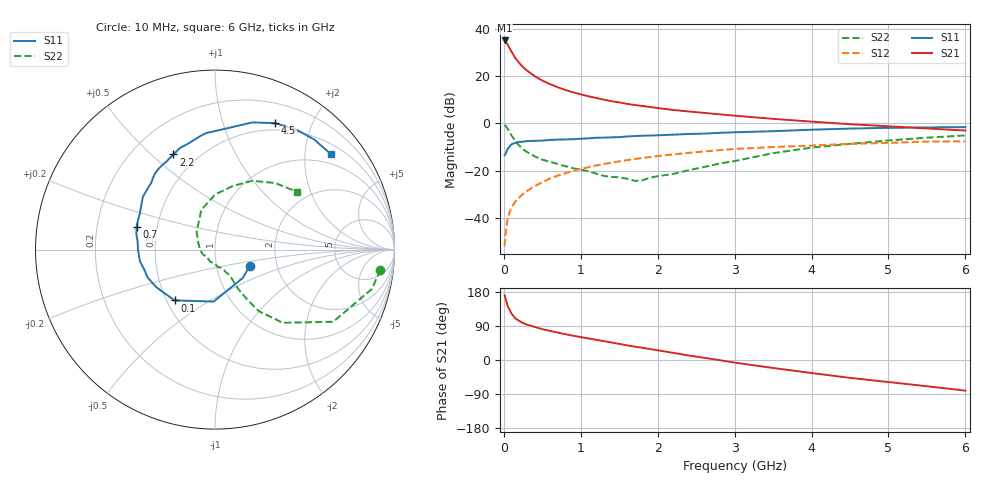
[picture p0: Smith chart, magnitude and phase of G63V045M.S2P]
! SIEMENS Small Signal Semiconductors
! BFG193
! Si NPN RF Bipolar Junction Transistor in SOT223
! VCE = 3 V  IC = 45 mA
! Common Emitter S-Parameters:  August  1996
# GHz  S  MA  R  50
!  f  S11  S21  S12  S22
! GHz  MAG  ANG  MAG  ANG  MAG  ANG  MAG  ANG
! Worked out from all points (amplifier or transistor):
!   36 points, 10 MHz to 6 GHz, reference 50 ohm
!   highest |S21| = 35.2 dB at 10 MHz (marker M1)
!   |S21| within 3 dB of that: start of sweep to 70.25 MHz
!   unconditionally stable (mu >= 1): 419.4 MHz to 2.427 GHz
!   at 250 MHz: K = 0.91, MSG = 26.9 dB, |S12| = -29.9 dB
!   at 1.4 GHz: K = 1.05, MAG = 11.7 dB, |S12| = -16.7 dB
!   at 6 GHz: K = 0.90, MSG = 2.3 dB, |S12| = -7.6 dB
!   S11 on the Smith chart (normalised r, x): 10 MHz: 1.45, -0.28; 100 MHz: 0.55, -0.36; 700 MHz: 0.38, +0.12; 2.2 GHz: 0.37, +0.59; 4.5 GHz: 0.42, +1.50; 6 GHz: 0.73, +2.60
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0.01  0.2138 -25.1  57.66 171.1  0.0025 82.6  0.9279 -7.0
0.02  0.2213 -45.4  55.79 163.3  0.0042 82.5  0.9011 -14.1
0.05  0.2896 -91.5  46.95 142.3  0.0099 70.2  0.7717 -31.4
0.1  0.3617 -128.5  33.24 122.4  0.0169 66.5  0.5558 -47.2
0.15  0.3886 -147.4  24.41 109.9  0.022 65.3  0.4198 -54.6
0.2  0.4062 -157.5  19.25 103.1  0.0269 66.3  0.3408 -56.9
0.25  0.4106 -165.1  15.7 97.6  0.0321 67.2  0.2828 -58.5
0.3  0.423 -170.8  13.27 93.4  0.037 68.6  0.25 -59.5
0.4  0.4284 -179.2  10.11 87.3  0.0468 68.5  0.2004 -59.9
0.5  0.4342 173.6  8.132 81.4  0.0568 67.6  0.171 -60.1
0.6  0.4475 168.5  6.834 76.8  0.0679 66.6  0.154 -61.6
0.7  0.4551 163.9  5.876 72.3  0.0781 65.5  0.1385 -64.4
0.9  0.4638 154.8  4.587 64.1  0.0991 61.8  0.1125 -68.9
1.1  0.4844 147.4  3.776 56.9  0.1184 58.3  0.0971 -80.4
1.3  0.5017 140.5  3.203 49.6  0.1384 54.2  0.0774 -92.2
1.6  0.5296 130.6  2.61 38.7  0.1669 47.5  0.0672 -120.5
2.2  0.5787 113.6  1.938 18.9  0.2212 33.8  0.0849 176.5
2.8  0.6323 98.6  1.566 -0.3  0.2724 19.8  0.1409 136.6
3.5  0.6859 82.7  1.254 -21.1  0.3166 2.4  0.2349 109.0
4.5  0.7799 64.6  0.965 -47.1  0.3698 -17.6  0.3694 74.1
5.5  0.8258 48.0  0.784 -69.3  0.4134 -40.8  0.5001 47.9
6  0.836 39.6  0.708 -80.8  0.4182 -54.1  0.5579 35.3
